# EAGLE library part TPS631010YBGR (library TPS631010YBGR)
Texas Instruments Source: Datasheet
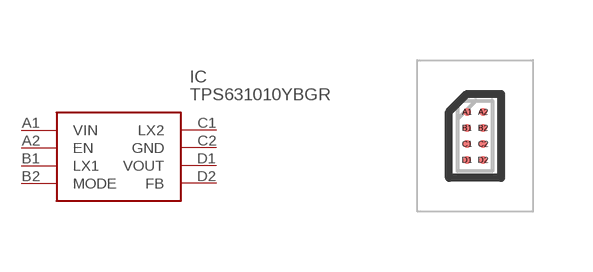
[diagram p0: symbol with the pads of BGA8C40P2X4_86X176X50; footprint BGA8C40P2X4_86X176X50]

Designator prefix IC

## TPS631010YBGR (Description: Texas Instruments; Height: 0.5mm; Manufacturer_Name: Texas Instruments; Manufacturer_Part_Number: TPS631010YBGR; Mouser_Part_Number: 595-TPS631010YBGR; Mouser_Price-Stock: https://www.mouser.co.uk/ProductDetail/Texas-Instruments/TPS631010YBGR?qs=rQFj71Wb1eUnypyc1JLtRA%3D%3D)  [BGA8C40P2X4_86X176X50]
A1  VIN
A2  EN
B1  LX1
B2  MODE
C1  LX2
C2  GND
D1  VOUT
D2  FB

## Footprint BGA8C40P2X4_86X176X50 (pad centres in mm)
YBG0008_2023
smd 0.2 x 0.2: A1 -0.2,0.6; A2 0.2,0.6; B1 -0.2,0.2; B2 0.2,0.2; C1 -0.2,-0.2; C2 0.2,-0.2; D1 -0.2,-0.6; D2 0.2,-0.6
